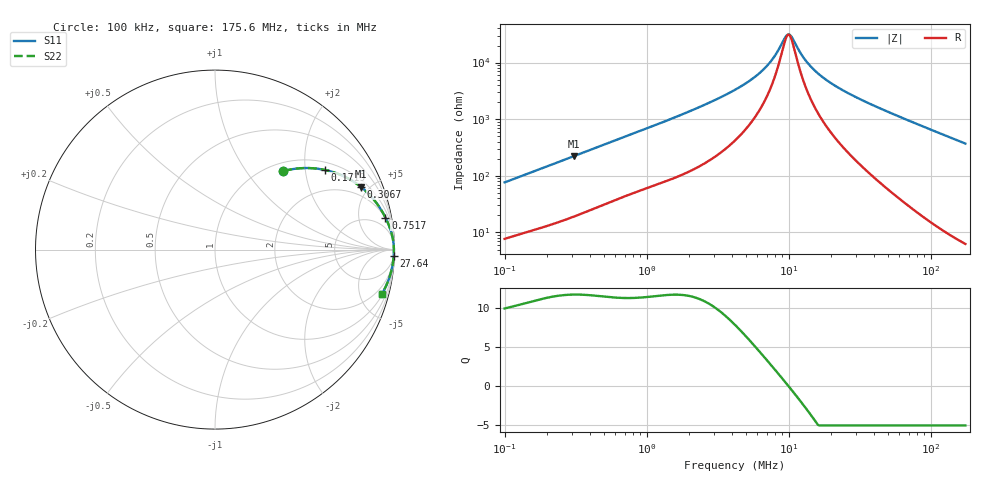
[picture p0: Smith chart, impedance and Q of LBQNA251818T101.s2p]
! LBQNA251818T101  S-PARAMETER MODEL  ( General Type )
! Model Generated by TAIYO YUDEN Corporation (http://www.ty-top.com)
! Version 1.0
! TAIYO YUDEN Control No. 191025NI43SB-FBB
! Copyright(c) 2019 TAIYO YUDEN CO.,LTD. All Rights Reserved.
! Product Description (link to TY-COMPAS)
! https://ds.yuden.co.jp/TYCOMPAS/or/detail?pn=LBQNA251818T101K&u=M
! Products Name : Inductors
! Characteristics :
!  Inductance : 100 uH , SRF(min) : 9.0 MHz , DC Resistance(max) : 2.73 Ohm
!  Rated Current : Saturation :60 mA , Temp Rise : 190 mA (20 degC)
!  Case Size : 2.5 x 1.8 / 0.098 x 0.071 [mm/inch] , Thickness : 1.8 / 0.071 [mm/inch]
!  (Conditions: Temperature = 25 degC , DC Bias Current/Voltage = 0A / 0V)
! External Node Assignments :
!  1  o---GGG---o  2
! GND o---------o GND
! Frequency Range : 0.1MHz  -  175.64884MHz  [ 402 STEP ]
# MHz S RI R 50
! Freq[MHz].  S11 Real  S11 Imag  S21 Real  S21 Imag  S12 Real  S12 Imag  S22 Real  S22 Imag
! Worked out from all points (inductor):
!   401 points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, 100 kHz to 175.6 MHz, reference 50 ohm
!   read as one part in series: L = 119 uH near 103.8 kHz
!   highest Q = 11.6 at 306.7 kHz (marker M1), where L = 115 uH
!   self-resonance near 9.896 MHz
!   S11 on the Smith chart (normalised r, x): 100 kHz: 1.15, +1.52; 171.9 kHz: 1.23, +2.54; 306.7 kHz: 1.38, +4.43; 751.7 kHz: 2, +10; 27.64 MHz: 5, -54; 175.6 MHz: 1.13, -7.42
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0.1  0.3809 0.4376  0.6191 -0.4376  0.6191 -0.4376  0.3809 0.4376
0.171885  0.6103 0.4442  0.3897 -0.4442  0.3897 -0.4442  0.6103 0.4442
0.306688  0.8115 0.3505  0.1885 -0.3505  0.1885 -0.3505  0.8115 0.3505
0.349525  0.8435 0.3229  0.1565 -0.3229  0.1565 -0.3229  0.8435 0.3229
0.498424  0.9071 0.2497  0.0929 -0.2497  0.0929 -0.2497  0.9071 0.2497
0.751717  0.9498 0.1783  0.0502 -0.1783  0.0502 -0.1783  0.9498 0.1783
1.221676  0.976 0.1155  0.024 -0.1155  0.024 -0.1155  0.976 0.1155
2.531099  0.9918 0.0554  0.00825 -0.0554  0.00825 -0.0554  0.9918 0.0554
4.270063  0.9953 0.029  0.00465 -0.029  0.00465 -0.029  0.9953 0.029
5.546217  0.9961 0.0189  0.00385 -0.0189  0.00385 -0.0189  0.9961 0.0189
6.811215  0.9965 0.0119  0.00348 -0.0119  0.00348 -0.0119  0.9965 0.0119
7.762576  0.9967 0.00775  0.00332 -0.00775  0.00332 -0.00775  0.9967 0.00775
9.356685  0.9968 0.00197  0.00319 -0.00197  0.00319 -0.00197  0.9968 0.00197
9.895935  0.9968 0.000263  0.00317 -0.000263  0.00317 -0.000263  0.9968 0.000263
10.46626  0.9968 -0.00145  0.00315 0.00145  0.00315 0.00145  0.9968 -0.00145
12.6156  0.9968 -0.00721  0.00316 0.00721  0.00316 0.00721  0.9968 -0.00721
14.64875  0.9968 -0.012  0.00324 0.012  0.00324 0.012  0.9968 -0.012
19.02669  0.9965 -0.0211  0.00352 0.0211  0.00352 0.0211  0.9965 -0.0211
27.64366  0.9956 -0.0367  0.00442 0.0367  0.00442 0.0367  0.9956 -0.0367
51.20104  0.9912 -0.0749  0.00881 0.0749  0.00881 0.0749  0.9912 -0.0749
96.62148  0.9756 -0.143  0.0244 0.143  0.0244 0.143  0.9756 -0.143
175.6488  0.9286 -0.2491  0.0714 0.2491  0.0714 0.2491  0.9286 -0.2491
